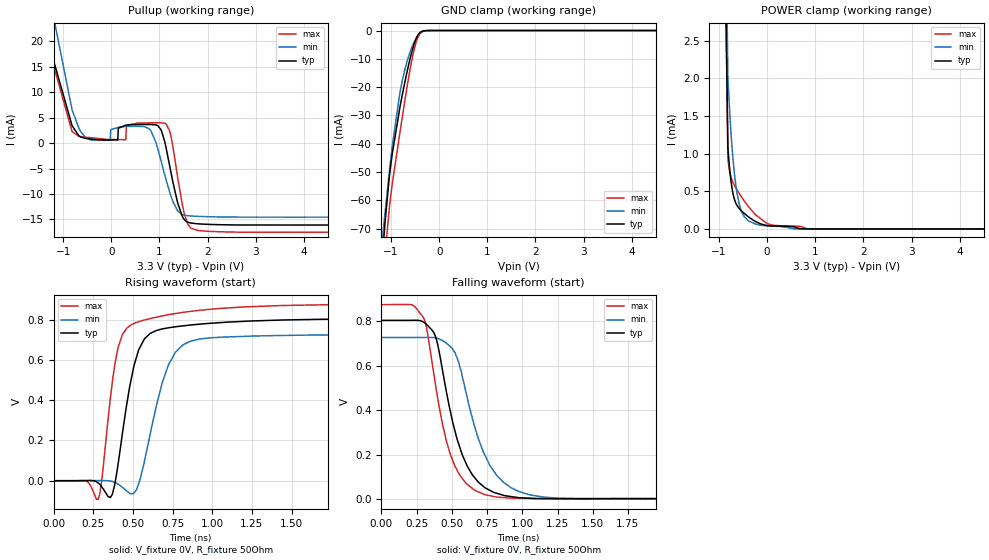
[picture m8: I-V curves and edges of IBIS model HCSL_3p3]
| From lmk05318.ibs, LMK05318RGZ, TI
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|   HCSL_3p3 Model
[Model]   HCSL_3p3
Model_type   Open_source
Polarity   Non-Inverting
Vmeas = 0.409
Vref = 0
Cref = 2pF
Rref = 50
|   typ   min   max
C_comp   1.41794E-12   1.36037E-12   1.45091E-12
| Where nom  PVT is Nominal Process, 3.3V, 27C
|   Fast PVT is Strong Process,  3.45V, -40C
|   Slow PVT is Weak Process,   3.15V, 125C
[Voltage Range]   3.3   3.15   3.45
|Junction Temperature
[Temperature Range]   27   125   -40
[Pullup Reference]   3.3   3.15   3.45
[Pulldown Reference]   0   0   0
[Power Clamp Reference]   3.3   3.15   3.45
[GND Clamp Reference]   0   0   0
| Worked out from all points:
|   GND clamp passes 1 mA (typ) near -0.41 V on its own axis
|   POWER clamp passes 1 mA (typ) near -0.80 V on its own axis
|   falling waveform, V_fixture 0V, R_fixture 50Ohm: 20-80 % time 185ps typ, 215ps min, 167ps max; typ from 0.803 V to 0 V
|   rising waveform, V_fixture 0V, R_fixture 50Ohm: 20-80 % time 112ps typ, 142ps min, 95.5ps max; typ from -0.001 V to 0.803 V
[GND Clamp]
|   Voltage   I(typ)   I(min)   I(max)
-3.3V     -1.225A    -1.029A    -1.515A
-1.181V   -80.15mA   -73.74mA   -92.54mA
-1.132V   -69.26mA   -65.41mA   -80.58mA
-1.122V   -67.19mA   -63.77mA   -78.45mA
-1.033V   -51.11mA   -49.44mA   -62.14mA
-973.5mV  -43.33mA   -40.6mA    -53.92mA
-815.1mV  -26.99mA   -21.86mA   -35.94mA
-765.6mV  -22.62mA   -17.58mA   -30.43mA
-528mV    -5.185mA   -4.26mA    -7.227mA
-438.9mV  -1.534mA   -1.654mA   -2.27mA
-349.8mV  -210.4uA   -427.7uA   -364.9uA
6.6V      0A         0A         0A
[Pullup]
|   Voltage   I(typ)   I(min)   I(max)
-3.3V     217.7mA    270.7mA    174.7mA
-1.518V   31.18mA    49.73mA    26.7mA
-1.35V    21.25mA    31.94mA    20.42mA
-815.1mV  3.451mA    6.573mA    2.261mA
-448.8mV  824.3uA    698uA      1.086mA
303.6mV   3.52mA     3.278mA    679uA
313.5mV   3.542mA    3.28mA     3.38mA
788.7mV   3.662mA    2.803mA    3.986mA
1.135V    -788.7uA   -7.131mA   3.809mA
1.383V    -11.88mA   -13.36mA   -6.963mA
1.66V     -15.73mA   -14.34mA   -16.78mA
6.6V      -16.11mA   -14.56mA   -17.54mA
[POWER Clamp]
|   Voltage   I(typ)   I(min)   I(max)
-3.3V     2.746A     3.266A     2.249A
-1.488V   31.11mA    34.76mA    35.04mA
-815.1mV  1.082mA    2.027mA    922.5uA
-775.5mV  776.3uA    1.532mA    752.1uA
-726mV    528.1uA    1.059mA    641.3uA
-627mV    314.2uA    482.9uA    520.1uA
-557.7mV  256.3uA    280uA      449.6uA
-478.5mV  207.7uA    164.7uA    374.7uA
-260.7mV  105.7uA    70.86uA    202.7uA
75.9mV    41.45uA    37.03uA    56.03uA
897.6mV   0A         127.3nA    190.6nA
6.6V      0A         0A         0A
[Ramp]
R_load = 50
|   typ   min   max
dV/dt_r   0.48208/1.12368e-10   0.435938/1.41774e-10   0.524597/9.54974e-11
dV/dt_f   0.482065/1.85341e-10   0.435889/2.15174e-10   0.524592/1.66827e-10
[Falling Waveform]
V_fixture = 0V
V_fixture_min = 0V
V_fixture_max = 0V
R_fixture = 50Ohm
C_fixture = 0F
|   Time   V(typ)   V(min)   V(max)
0s        803mV      726.3mV    873.9mV
291.2ps   798mV      726.4mV    822.5mV
370.9ps   749.2mV    725.8mV    566.9mV
433.9ps   577.6mV    712.3mV    335mV
521.5ps   307.5mV    658.5mV    149mV
609.2ps   148.6mV    455.6mV    67.24mV
733.8ps   52.41mV    198.6mV    20.6mV
919.4ps   12mV       51.91mV    4.996mV
1.262ns   1.836mV    4.429mV    3.589mV
5ns       -409.5uV   -214.2uV   -402.1uV
[Rising Waveform]
V_fixture = 0V
V_fixture_min = 0V
V_fixture_max = 0V
R_fixture = 50Ohm
C_fixture = 0F
|   Time   V(typ)   V(min)   V(max)
0s        -566.5uV   -359.4uV   -592.3uV
205.1ps   -16.36uV   106.1uV    -1.393mV
281.9ps   -11.73mV   280.5uV    -92.97mV
358.4ps   -84.27mV   -2.454mV   412.5mV
433.9ps   233.8mV    -33.22mV   726.5mV
521.9ps   612mV      -46mV      786.5mV
662.1ps   749.8mV    416.9mV    815.8mV
767.8ps   765.2mV    638.7mV    831.1mV
979.6ps   782.3mV    709.7mV    851.7mV
5ns       802.9mV    726.2mV    873.7mV
